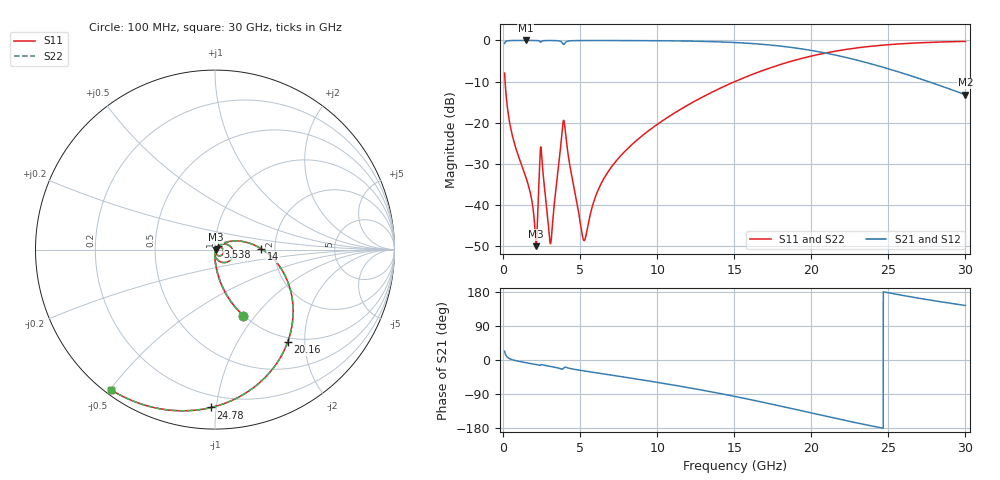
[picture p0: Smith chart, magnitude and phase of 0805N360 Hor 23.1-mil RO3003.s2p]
# GHz S MA R 50
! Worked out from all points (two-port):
!   3201 points, 100 MHz to 30 GHz, reference 50 ohm
!   highest |S21| = -0.01 dB at 1.464 GHz (marker M1); lowest = -13.2 dB at 30 GHz (marker M2)
!   |S21| within 3 dB of the highest: start of sweep to 20.85 GHz
!   lowest |S11| = -50.0 dB at 2.156 GHz (marker M3), VSWR 1.01, Z = 50.3 - j0.129 ohm
!   |S11| at or under -10 dB: 131.2 MHz to 15.05 GHz (14.91 GHz wide, 197 % of centre)
!   |S22| runs from -50.0 to -0.2 dB; largest |S21 - S12| = 0
!   S11 on the Smith chart (normalised r, x): 100 MHz: 0.99, -0.87; 3.538 GHz: 1.03, +0.04; 14 GHz: 1.69, +0.02; 20.16 GHz: 0.92, -1.66; 24.78 GHz: 0.12, -0.97; 30 GHz: 0.02, -0.50
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0.1  0.4008 -66.9  0.9158 23.1  0.9158 23.1  0.4008 -66.9
0.5578437  0.07586 -88.3  0.9965 1.3  0.9965 1.3  0.07586 -88.3
1.464187  0.02219 -94.1  0.9986 -6.9  0.9986 -6.9  0.02219 -94.1
2.155625  0.00316 -23.9  0.9968 -11.9  0.9968 -11.9  0.00316 -23.9
2.463969  0.0496 -36.5  0.9544 -12.5  0.9544 -12.5  0.0496 -36.5
3.061969  0.00341 -26.0  0.9965 -16.9  0.9965 -16.9  0.00341 -26.0
3.183438  0.005129 27.3  0.9963 -17.8  0.9963 -17.8  0.005129 27.3
3.5385  0.02323 48.6  0.9914 -20.8  0.9914 -20.8  0.02323 48.6
3.828156  0.0787 19.4  0.9414 -24.2  0.9414 -24.2  0.0787 19.4
3.977656  0.09962 -42.5  0.9073 -19.7  0.9073 -19.7  0.09962 -42.5
5.089563  0.004892 -63.7  0.9958 -27.8  0.9958 -27.8  0.004892 -63.7
5.323156  0.00386 -7.9  0.9962 -29.3  0.9962 -29.3  0.00386 -7.9
6.023937  0.01303 42.3  0.9965 -33.7  0.9965 -33.7  0.01303 42.3
6.986344  0.0282 44.1  0.9963 -39.6  0.9963 -39.6  0.0282 44.1
10.06978  0.0973 28.4  0.9912 -59.4  0.9912 -59.4  0.0973 28.4
14.0035  0.2577 1.1  0.9607 -87.8  0.9607 -87.8  0.2577 1.1
15.05  0.3165 -7.2  0.9426 -96.2  0.9426 -96.2  0.3165 -7.2
20.03956  0.6478 -50.8  0.7535 -140.1  0.7535 -140.1  0.6478 -50.8
20.16103  0.6556 -51.9  0.7467 -141.2  0.7467 -141.2  0.6556 -51.9
24.77684  0.88 -91.4  0.4649 179.1  0.4649 179.1  0.88 -91.4
25.01978  0.8874 -93.3  0.4508 177.3  0.4508 177.3  0.8874 -93.3
30  0.9728 -126.6  0.2186 143.9  0.2186 143.9  0.9728 -126.6
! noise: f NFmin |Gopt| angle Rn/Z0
0.1  0.0004675  0.8707  0.7965  0.0007786
3.417  0.01028  0.8073  18.85  0.01081
6.743  0.0109  0.6742  36.63  0.005835
10.06  0.01442  0.6486  53.25  0.006297
13.39  0.01891  0.6537  68.74  0.007226
16.7  0.02453  0.6744  83.1  0.008373
20.03  0.03203  0.7068  96.64  0.009846
23.35  0.04263  0.7489  109.6  0.01183
26.67  0.05884  0.7984  122.4  0.01459
30  0.08574  0.8511  135.3  0.01839
